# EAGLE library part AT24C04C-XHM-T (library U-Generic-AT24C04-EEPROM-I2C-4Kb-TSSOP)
EEPROM with I2C interface
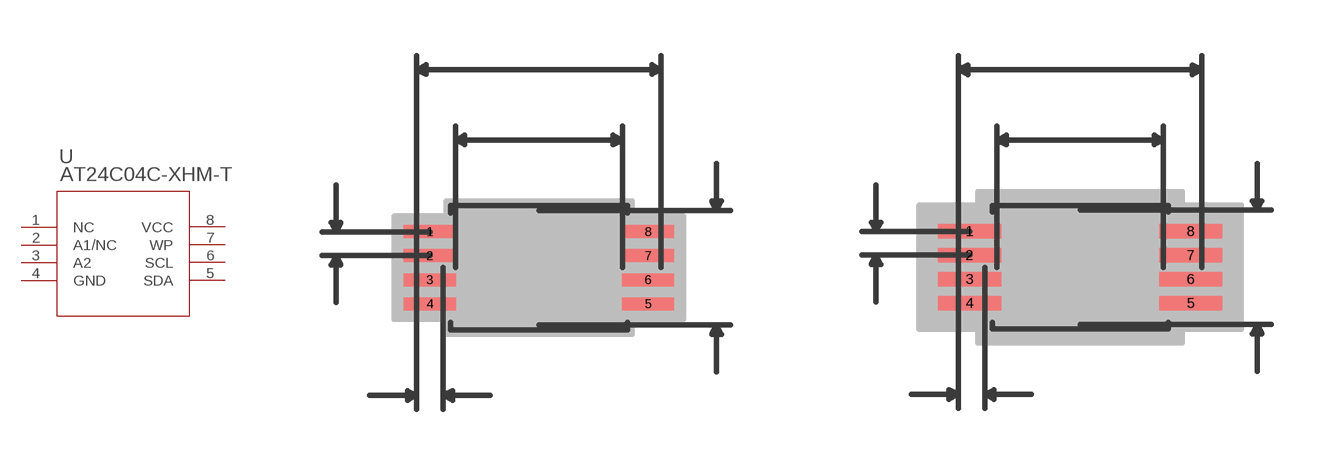
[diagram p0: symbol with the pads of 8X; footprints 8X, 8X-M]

Designator prefix U

## AT24C04C-XHM-T (MANUFACTURER_PART_NUMBER: AT24C04CXHMT; VENDOR: Atmel)  [8X]
1  NC  nc
2  A1/NC
3  A2  in
4  GND  pwr
5  SDA  pas
6  SCL  in
7  WP  pas
8  VCC  pwr

## AT24C04C-XHM-T8X-M (MANUFACTURER_PART_NUMBER: AT24C04CXHMT; VENDOR: Atmel)  [8X-M]
Pads as for 8X

## AT24C04C-XHM-T8X-L (MANUFACTURER_PART_NUMBER: AT24C04CXHMT; VENDOR: Atmel)  [8X-L]
Pads as for 8X

## Footprint 8X (pad centres in mm)
smd 1.411 x 0.351: 1 -2.95,0.975; 2 -2.95,0.325; 3 -2.95,-0.325; 4 -2.95,-0.975; 5 2.95,-0.975; 6 2.95,-0.325; 7 2.95,0.325; 8 2.95,0.975

## Footprint 8X-M (pad centres in mm)
smd 1.716 x 0.402: 1 -3.001,0.975; 2 -3.001,0.325; 3 -3.001,-0.325; 4 -3.001,-0.975; 5 3.001,-0.975; 6 3.001,-0.325; 7 3.001,0.325; 8 3.001,0.975

## Footprint 8X-L (pad centres in mm)
smd 1.106 x 0.3: 1 -2.899,0.975; 2 -2.899,0.325; 3 -2.899,-0.325; 4 -2.899,-0.975; 5 2.899,-0.975; 6 2.899,-0.325; 7 2.899,0.325; 8 2.899,0.975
